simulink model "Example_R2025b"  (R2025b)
settings: Solver=VariableStepAuto  StartTime=0.0  StopTime=100  RelTol=1e-3
libraries: MotionSystems_Simulink_R2025b x2

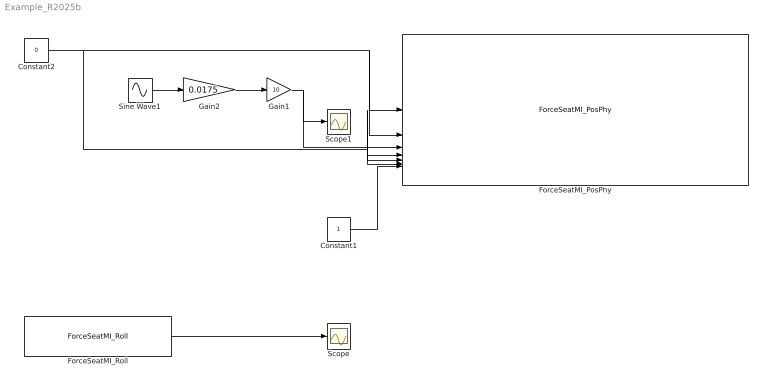
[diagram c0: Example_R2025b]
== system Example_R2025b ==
  Constant1 : Constant  OutDataTypeStr=int32
  Constant2 : Constant  Value=0
  ForceSeatMI_PosPhy : MotionSystems_Simulink_R2025b/ForceSeatMI_PosPhy  SampleTime=-1
  ForceSeatMI_Roll : MotionSystems_Simulink_R2025b/ForceSeatMI_Roll  SampleTime=-1
  Gain1 : Gain  Gain=10
  Gain2 : Gain  Gain=0.0175
  Scope : Scope
  Scope1 : Scope
  Sine Wave1 : Sin  SampleTime=0.01
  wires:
  Constant1/1 -> ForceSeatMI_PosPhy/7
  Constant2/1 -> ForceSeatMI_PosPhy/2, ForceSeatMI_PosPhy/1, ForceSeatMI_PosPhy/6, ForceSeatMI_PosPhy/5, ForceSeatMI_PosPhy/4
  Sine Wave1/1 -> Gain2/1
  Gain2/1 -> Gain1/1
  Gain1/1 -> ForceSeatMI_PosPhy/3, Scope1/1
  ForceSeatMI_Roll/1 -> Scope/1
